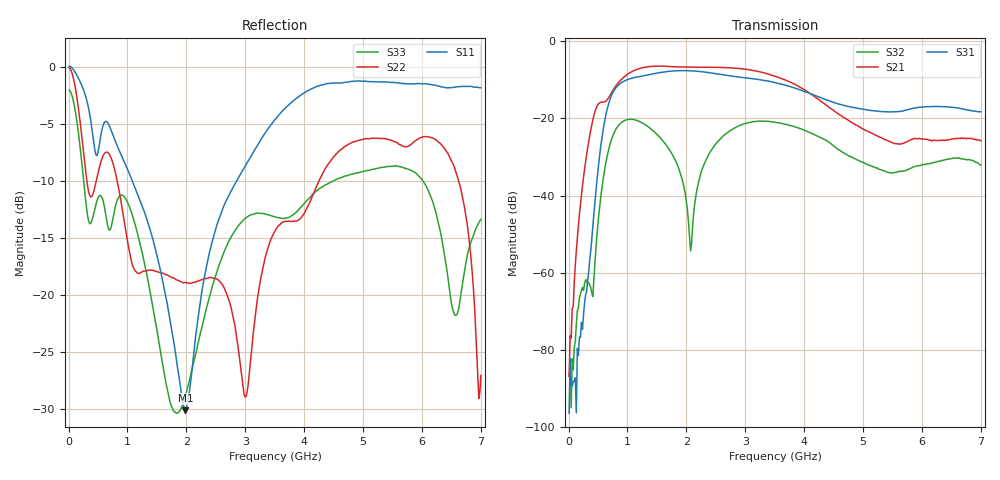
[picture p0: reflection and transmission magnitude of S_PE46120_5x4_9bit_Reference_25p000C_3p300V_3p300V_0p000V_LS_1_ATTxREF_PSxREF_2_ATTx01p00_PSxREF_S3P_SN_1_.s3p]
! Device ID: PE46120_5x4_9bit_Reference
! Device ID: PE46120_5x4_9bit_Reference
! File Path: z:\PE46120_5x4_9bit_Reference\MPAC_Yi\new_12port\25p000C\3p300\LS_1_ATTxREF_PSxREF_2_ATTx01p00_PSxREF\PE46120_5x4_9bit_Reference_25p000C_3p300V_3p300V_0p000V_LS_1_ATTxREF_PSxREF_2_ATTx01p00_PSxREF_S3P_SN_1_.s3p
! Serial: 1
! Lot:
! Temp: 25.000C
! VDD: 3.300
! VSS: 0.000
! Control_Hi: 3.300
! Control_Lo: 0.000
! Logic State: LS_1_ATTxREF_PSxREF_2_ATTx01p00_PSxREF
! Port 1: RFin
! Port 2: RFout1
! Port 3: RFout2
! ThroughPath:1-3
! IDD: -0.0005399574
! ISS: 0
! Comment:
#  Hz  S  RI  R  50
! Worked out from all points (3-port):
!   401 points, 10 MHz to 7 GHz, reference 50 ohm
!   strongest paths, dB at 10 MHz, 1.758 GHz, 3.505 GHz, 5.253 GHz, 7 GHz:
!     S31: -96.5, -7.7, -10.7, -18.1, -18.3
!     S21: -86.9, -6.5, -9.0, -24.6, -25.8
!     S32: -86.9, -29.2, -20.9, -33.1, -32.1
!   lowest |S11| = -30.1 dB at 1.985 GHz (marker M1), VSWR 1.06, Z = 52.8 + j1.6 ohm
!   |S11| at or under -10 dB: 1.082 GHz to 2.854 GHz (1.772 GHz wide, 90.1 % of centre)
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1e7  1.001 -0.115  0.000102 -1.04e-05  -0.000101 6.27e-05
     4.54e-05 7.24e-07  0.9875 -0.0964  5.63e-05 2.87e-05
     -1.44e-05 -4.33e-06  -4.4e-05 9.49e-06  0.7876 -0.0758
2.5465e8  -0.5336 -0.5874  -0.016 -0.00579  0.000128 0.000259
          -0.0163 -0.00595  -0.3279 -0.268  -0.000242 0.000678
          0.000118 0.000262  -0.000154 0.000571  -0.2455 -0.2043
4.81825e8  -0.3984 -0.0877  -0.0453 0.1341  0.0151 0.00302
           -0.0458 0.1359  0.1908 0.2635  -0.00204 0.00214
           0.0154 0.00303  -0.00208 0.00226  0.1766 0.1881
9.5365e8  -0.2778 0.2576  0.3393 -0.0704  -0.0814 0.2935
          0.3431 -0.0715  -0.0536 -0.1963  -0.0449 0.0815
          -0.082 0.2971  -0.0452 0.0827  0.0943 -0.2509
1.984675e9  0.0272 0.0152  -0.3719 0.2676  -0.2519 -0.3268
            -0.3759 0.2713  -0.0913 0.0663  0.000982 0.0102
            -0.2558 -0.3302  0.00106 0.0102  -0.0351 0.00825
2.806e9  -0.0752 -0.2904  0.4354 0.0956  -0.0874 0.3364
         0.4407 0.0961  0.0726 -0.0262  0.0117 0.0725
         -0.0874 0.341  0.012 0.0734  0.0748 0.172
3.505e9  -0.4368 -0.3925  -0.0886 -0.3376  0.2849 0.0471
         -0.0899 -0.3417  0.0621 0.1797  0.0104 -0.0879
         0.2887 0.0472  0.0106 -0.089  0.1712 -0.1375
4.605925e9  -0.8482 0.0526  -0.0091 0.1095  -0.0652 -0.1357
            -0.00915 0.1103  -0.4024 0.152  0.0262 0.0273
            -0.0667 -0.1374  0.0269 0.0279  -0.1931 0.2618
6.248575e9  -0.376 0.7377  0.0407 -0.0313  -0.0178 0.1402
            0.0411 -0.0317  0.4671 -0.0918  -0.0261 -0.0063
            -0.0177 0.1421  -0.0265 -0.00655  0.1909 -0.1149
7e9  -0.1167 0.801  -0.0291 -0.0416  0.1094 0.0499
     -0.0297 -0.0419  -0.0404 0.018  0.0224 0.00863
     0.1114 0.0501  0.0232 0.00872  0.135 0.1663
